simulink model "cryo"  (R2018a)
settings: Solver=ode45  StartTime=0.0  StopTime=10.0  RelTol=1e-3  EnableMultiTasking=on

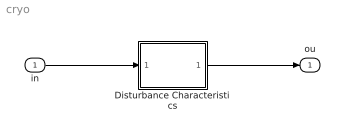
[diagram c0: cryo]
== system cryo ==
  in : Inport
  Disturbance Characteristics : Subsystem
  ou : Outport
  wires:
  in/1 -> Disturbance Characteristics/1(in)
  Disturbance Characteristics/1(ou) -> ou/1

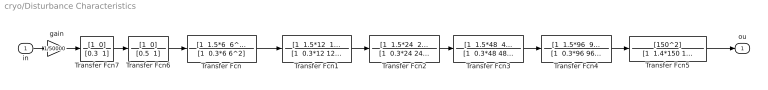
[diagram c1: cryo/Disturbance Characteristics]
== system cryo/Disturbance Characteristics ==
  in : Inport
  Transfer Fcn : TransferFcn  Numerator="[1  1.5*6  6^2]"  Denominator="[1  0.3*6 6^2]"
  Transfer Fcn1 : TransferFcn  Numerator="[1  1.5*12  12^2]"  Denominator="[1  0.3*12 12^2]"
  Transfer Fcn2 : TransferFcn  Numerator="[1  1.5*24  24^2]"  Denominator="[1  0.3*24 24^2]"
  Transfer Fcn3 : TransferFcn  Numerator="[1  1.5*48  48^2]"  Denominator="[1  0.3*48 48^2]"
  Transfer Fcn4 : TransferFcn  Numerator="[1  1.5*96  96^2]"  Denominator="[1  0.3*96 96^2]"
  Transfer Fcn5 : TransferFcn  Numerator=[150^2]  Denominator="[1  1.4*150 150^2]"
  Transfer Fcn6 : TransferFcn  Numerator="[1  0]"  Denominator="[0.5  1]"
  Transfer Fcn7 : TransferFcn  Numerator="[1  0]"  Denominator="[0.3  1]"
  gain : Gain  Gain=1/50000
  ou : Outport
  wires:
  in/1 -> gain/1
  Transfer Fcn/1 -> Transfer Fcn1/1
  Transfer Fcn1/1 -> Transfer Fcn2/1
  Transfer Fcn2/1 -> Transfer Fcn3/1
  Transfer Fcn3/1 -> Transfer Fcn4/1
  gain/1 -> Transfer Fcn7/1
  Transfer Fcn4/1 -> Transfer Fcn5/1
  Transfer Fcn5/1 -> ou/1
  Transfer Fcn6/1 -> Transfer Fcn/1
  Transfer Fcn7/1 -> Transfer Fcn6/1
